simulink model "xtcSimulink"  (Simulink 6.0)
settings: Solver=ode45  StartTime=0.0  StopTime=100  RelTol=1e-3

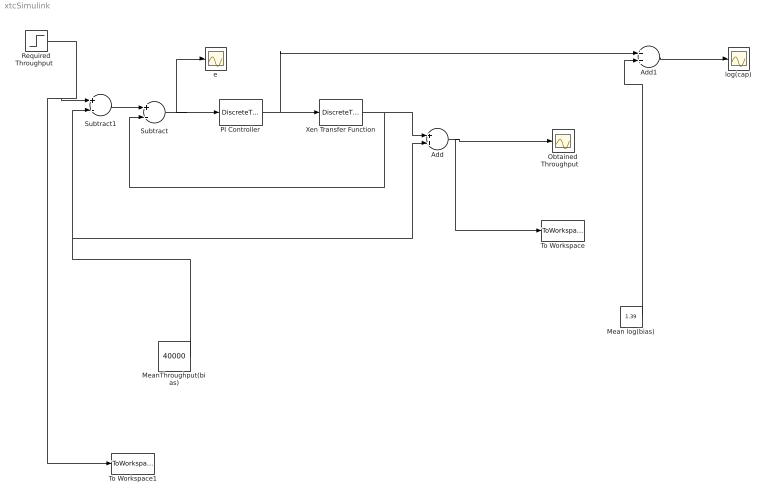
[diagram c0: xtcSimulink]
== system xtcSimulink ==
  Add : Sum  OutScaling=2^-10
  Add1 : Sum  OutScaling=2^-10
  Mean log(bias) : Constant  Value=1.39
  MeanThroughput(bias) : Constant  Value=40000
  "Obtained Throughput   " : Scope
  PI Controller : DiscreteTransferFcn  Numerator=[0.000018736 -0.000003422]  Denominator=[1 -1]  SampleTime=-1
  "Required Throughput  " : Step  Time=50  After=20000  SampleTime=1
  Subtract : Sum  Inputs=+-  OutScaling=2^-10
  Subtract1 : Sum  Inputs=+-  OutScaling=2^-10
  To Workspace : ToWorkspace  VariableName=obtainedThrouput  SampleTime=-1  SaveFormat=Array
  To Workspace1 : ToWorkspace  VariableName=requiredThroughput  SampleTime=-1  SaveFormat=Array
  Xen Transfer Function : DiscreteTransferFcn  Numerator=[32259]  Denominator=[1 -0.0915]  SampleTime=-1
  e : Scope
  log(cap) : Scope
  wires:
  Xen Transfer Function/1 -> Add/1, Subtract/2
  Subtract/1 -> e/1, PI Controller/1
  Subtract1/1 -> Subtract/1
  "Required Throughput  "/1 -> Subtract1/1, To Workspace1/1
  MeanThroughput(bias)/1 -> Subtract1/2, Add/2
  Add/1 -> "Obtained Throughput   "/1, To Workspace/1
  Mean log(bias)/1 -> Add1/2
  Add1/1 -> log(cap)/1
  PI Controller/1 -> Xen Transfer Function/1, Add1/1
